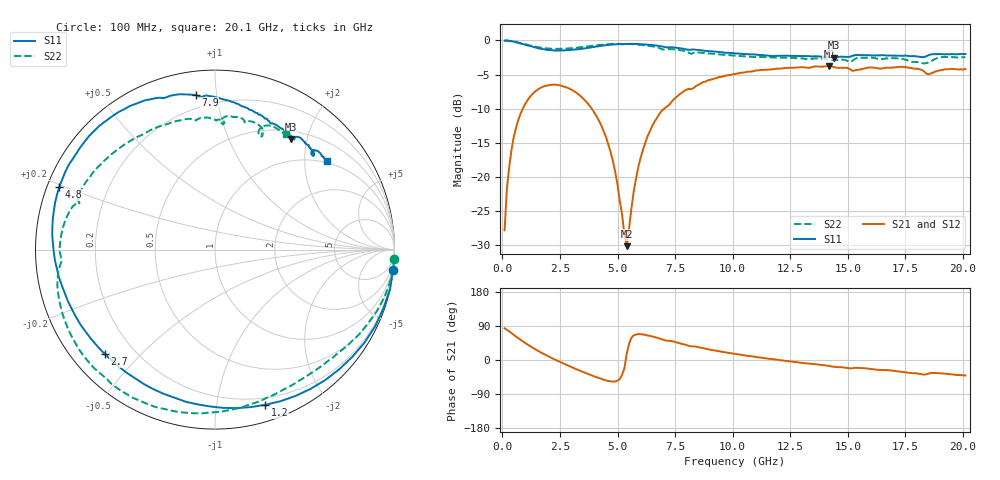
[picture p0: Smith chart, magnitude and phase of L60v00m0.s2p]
!  Infineon Technologies AG
! BFR380L3 Vierpol-Parameter eines
! 2PORT S-Parameters:  15. November 2001
#  GHz  S  MA  R  50
! f  S11  S21  S12  S22
! GHz  Mag  Ang  Mag  Ang  Mag  Ang  Mag  Ang
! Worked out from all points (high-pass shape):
!   201 points, 100 MHz to 20.1 GHz, reference 50 ohm
!   highest |S21| = -3.73 dB at 14.2 GHz (marker M1); lowest = -30.1 dB at 5.4 GHz (marker M2)
!   |S21| within 3 dB of the highest: 1.795 GHz to 2.655 GHz (860.8 MHz wide, 38.7 % of centre); 8.383 GHz to end of sweep
!   lowest |S11| = -2.5 dB at 14.4 GHz (marker M3), VSWR 6.90, Z = 31.2 + j86.7 ohm
!   |S11| at or under -10 dB: nowhere
!   |S22| runs from -3.4 to 0.0 dB; largest |S21 - S12| = 0.013
!   S11 on the Smith chart (normalised r, x): 100 MHz: 1, -17; 1.2 GHz: 0.14, -1.37; 2.7 GHz: 0.10, -0.39; 4.8 GHz: 0.03, +0.19; 7.9 GHz: 0.12, +0.87; 20.1 GHz: 0.96, +2.58
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0.1  0.9964 -6.6  0.04073 83.7  0.04088 84.6  1.001 -3.1
0.2  0.9999 -12.9  0.08207 79.8  0.08214 80.1  0.9985 -6.1
0.5  0.9811 -31.9  0.1973 66.0  0.1966 65.9  0.9812 -15.1
0.9  0.9408 -55.7  0.3192 48.7  0.3202 48.5  0.9458 -25.9
1.2  0.909 -72.0  0.3863 36.8  0.3869 36.7  0.9188 -33.4
1.8  0.8632 -100.9  0.4612 15.9  0.4609 15.9  0.8808 -46.6
2.7  0.8461 -136.6  0.4582 -10.5  0.46 -10.3  0.8703 -65.9
3.5  0.8712 -163.8  0.3771 -31.6  0.3778 -31.2  0.8966 -84.5
4.3  0.9149 172.1  0.2375 -49.8  0.2399 -49.7  0.9296 -105.4
4.8  0.9354 158.1  0.1308 -57.0  0.133 -57.2  0.9441 -119.1
5.4  0.9423 142.8  0.03112 16.2  0.03201 12.5  0.9433 -135.5
5.9  0.9408 131.0  0.1177 68.6  0.1201 67.7  0.9334 -149.1
6.3  0.9314 122.8  0.1982 64.5  0.1996 64.5  0.917 -159.7
6.8  0.9112 113.2  0.2864 57.4  0.2892 56.4  0.8811 -172.2
7.9  0.8683 97.2  0.4272 41.0  0.4305 40.1  0.839 165.4
10.1  0.8031 76.4  0.5678 16.3  0.566 15.3  0.7739 131.6
13.5  0.7659 58.3  0.642 -10.7  0.6319 -10.9  0.7344 97.1
14.2  0.7533 55.4  0.6509 -15.8  0.6392 -16.3  0.7269 90.8
14.4  0.7467 55.4  0.6381 -17.9  0.6334 -18.1  0.72 89.5
16.8  0.7778 47.0  0.6309 -27.2  0.6234 -27.5  0.7414 74.7
18.4  0.7658 45.4  0.5725 -37.7  0.5667 -37.8  0.6818 69.0
20.1  0.7966 38.1  0.6183 -40.7  0.6102 -40.8  0.754 58.6
